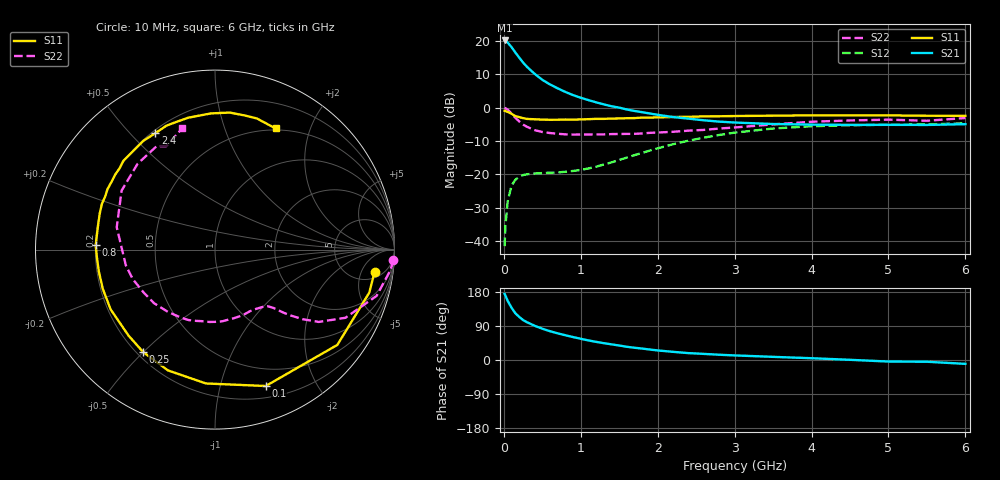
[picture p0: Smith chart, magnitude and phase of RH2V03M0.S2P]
! SIEMENS Small Signal Semiconductors
! BFR106
! Si NPN RF Bipolar Junction Transistor in SOT23
! VCE = 2 V  IC = 3 mA
! Common Emitter S-Parameters:  August  1996
# GHz  S  MA  R  50
!  f  S11  S21  S12  S22
! GHz  MAG  ANG  MAG  ANG  MAG  ANG  MAG  ANG
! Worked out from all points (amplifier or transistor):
!   36 points, 10 MHz to 6 GHz, reference 50 ohm
!   highest |S21| = 20.2 dB at 10 MHz (marker M1)
!   |S21| within 3 dB of that: start of sweep to 130.6 MHz
!   unconditionally stable (mu >= 1): 699.9 MHz to 2.17 GHz; 3.711 GHz to end of sweep
!   at 250 MHz: K = 0.39, MSG = 16.9 dB, |S12| = -20.2 dB
!   at 1.4 GHz: K = 1.24, MAG = 5.5 dB, |S12| = -16.4 dB
!   at 6 GHz: K = 1.02, MAG = -1.1 dB, |S12| = -4.7 dB
!   S11 on the Smith chart (normalised r, x): 10 MHz: 7, -9; 100 MHz: 0.31, -1.39; 250 MHz: 0.22, -0.50; 800 MHz: 0.20, +0.02; 2.4 GHz: 0.21, +0.59; 6 GHz: 0.48, +1.51
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0.01  0.8979 -7.9  10.25 174.4  0.0083 85.7  0.9955 -3.4
0.02  0.8923 -15.6  10.2 170.3  0.0164 84.0  0.9834 -6.8
0.05  0.8641 -37.9  9.536 156.0  0.0393 69.8  0.9363 -16.0
0.1  0.8109 -69.6  8.147 138.0  0.0672 55.0  0.82 -27.6
0.15  0.7475 -93.9  6.749 123.2  0.0828 44.1  0.7044 -34.9
0.2  0.7223 -111.3  5.662 113.6  0.0914 38.0  0.6223 -38.5
0.25  0.697 -125.1  4.777 105.5  0.0972 33.3  0.5578 -41.1
0.3  0.6794 -135.2  4.125 99.8  0.0999 31.3  0.5171 -42.7
0.4  0.6702 -150.2  3.233 90.4  0.1026 28.6  0.4604 -44.9
0.5  0.6623 -160.8  2.627 82.6  0.1041 28.4  0.4314 -47.0
0.6  0.6586 -169.4  2.238 76.0  0.1056 29.7  0.4164 -49.9
0.8  0.665 177.9  1.726 65.3  0.109 35.2  0.3978 -57.1
1.1  0.6729 162.6  1.3 51.6  0.1222 45.9  0.3961 -69.8
1.6  0.6956 143.1  0.94 34.9  0.1783 58.0  0.4044 -94.5
2.2  0.7257 123.3  0.724 21.5  0.2827 56.4  0.4348 -126.9
2.4  0.7286 117.2  0.685 18.2  0.3198 53.6  0.4522 -138.6
3  0.7499 101.5  0.599 12.1  0.4219 42.0  0.5044 -169.9
3.5  0.7592 91.7  0.569 8.3  0.4868 31.4  0.5614 167.2
4.5  0.7654 77.5  0.552 0.5  0.5448 12.2  0.6438 132.1
5  0.767 72.3  0.553 -4.1  0.5547 4.7  0.6617 119.4
5.5  0.7573 67.0  0.551 -4.6  0.5616 1.3  0.6369 115.2
6  0.755 63.4  0.566 -10.2  0.5837 -6.1  0.7002 105.1
